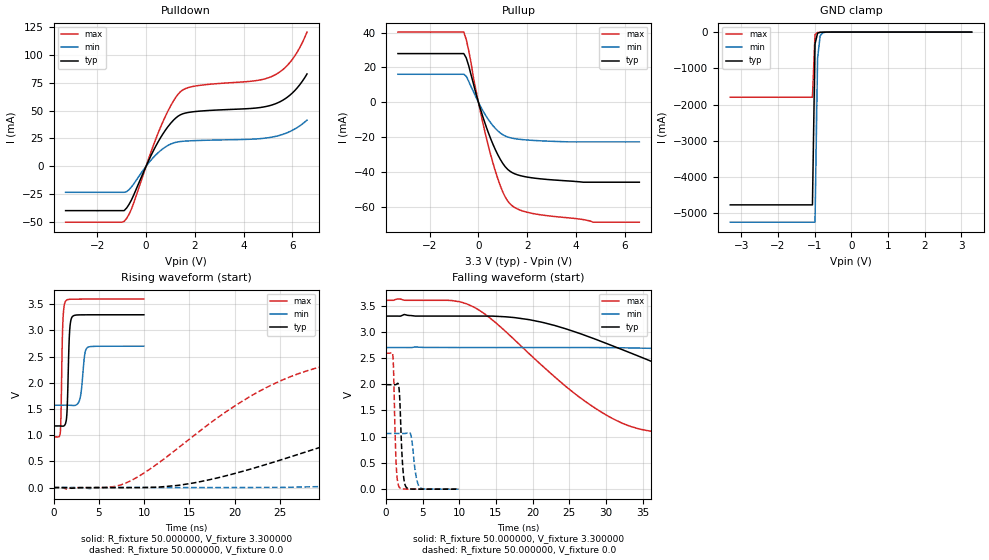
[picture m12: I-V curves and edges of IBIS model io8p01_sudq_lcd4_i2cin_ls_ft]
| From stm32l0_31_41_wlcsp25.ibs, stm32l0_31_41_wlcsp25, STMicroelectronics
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|   Model io8p01_sudq_lcd4_i2cin_ls_ft
[Model]  io8p01_sudq_lcd4_i2cin_ls_ft
Model_type I/O
Polarity   Non-Inverting
Enable   Active-Low
Vinl =   0.990000V
Vinh =   2.310000V
Vmeas =  1.650000V
Cref =   50.000000pF
Rref =   100.000000M
Vref =   0.0V
C_comp   2.499500pF   2.460800pF   2.557800pF
[Temperature Range]   25.000000   0.125000k   -40.000000
[Pullup Reference]   3.300000V   2.700000V   3.600000V
[Pulldown Reference]   0.0V   0.0V   0.0V
[POWER Clamp Reference]   3.300000V   2.700000V   3.600000V
[GND Clamp Reference]   0.0V   0.0V   0.0V
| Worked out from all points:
|   slope of the pulldown table from 0 to 0.495 V, typ, clamps not added: 22.6 ohm
|   slope of the pullup table from 0 to 0.495 V, typ, clamps not added: 23.9 ohm
|   GND clamp passes 1 mA (typ) near -0.64 V on its own axis
|   rising waveform, R_fixture 50.000000, V_fixture 3.300000: 20-80 % time 216ps typ, 364ps min, 176ps max; typ from 1.18 V to 3.3 V
|   rising waveform, R_fixture 50.000000, V_fixture 0.0: 20-80 % time 27.1ns typ, 59.7ns min, 13.6ns max; typ from 0 V to 1.99 V
|   falling waveform, R_fixture 50.000000, V_fixture 3.300000: 20-80 % time 24.2ns typ, 53.5ns min, 13.3ns max; typ from 3.3 V to 1.18 V
|   falling waveform, R_fixture 50.000000, V_fixture 0.0: 20-80 % time 383ps typ, 552ps min, 305ps max; typ from 1.99 V to 0 V
[Pulldown]
|Voltage   I(typ)   I(min)   I(max)
-3.3V     -39.83mA   -23.37mA   -50.2mA
-900mV    -39.83mA   -23.37mA   -49.53mA
-600mV    -30.28mA   -18.59mA   -38.45mA
500mV     22.11mA    12.28mA    30.1mA
1V        38.33mA    19.81mA    53.88mA
1.4V      46.1mA     22.18mA    66.72mA
2V        49.07mA    23.01mA    71.93mA
4.4V      52.05mA    24.38mA    76.53mA
5.2V      55.25mA    26.3mA     81.02mA
5.6V      59.18mA    28.57mA    86.57mA
6V        65.78mA    32.24mA    95.96mA
6.6V      82.83mA    41.41mA    120.4mA
[Pullup]
|Voltage   I(typ)   I(min)   I(max)
-3.3V     27.97mA    16.08mA    40.34mA
-600mV    27.97mA    16.08mA    40.34mA
-400mV    21.06mA    12.09mA    29.9mA
-200mV    10.4mA     5.946mA    13.84mA
200mV     -9.115mA   -5.294mA   -12.98mA
600mV     -24.29mA   -13.56mA   -35.12mA
1V        -35.2mA    -18.69mA   -51.63mA
1.2V      -38.62mA   -20mA      -56.79mA
1.4V      -40.6mA    -20.72mA   -59.71mA
2.2V      -43.48mA   -21.92mA   -63.91mA
4.7V      -46.01mA   -22.8mA    -69mA
6.6V      -46.01mA   -22.8mA    -69mA
[GND_clamp]
|Voltage   I(typ)   I(min)   I(max)
-3.3V     -4.766A    -5.244A    -1.797A
-1.06V    -4.766A    -5.244A    -1.797A
-990mV    -326.4mA   -5.244A    -67.85mA
-920mV    -28.83mA   -721.7mA   -11.08mA
-850mV    -6.686mA   -104.1mA   -6.707mA
-780mV    -3.552mA   -17.28mA   -4.326mA
-500mV    -59.41uA   -172uA     -34.91uA
3.28V     0A         0A         0A
[POWER_clamp]
|Voltage   I(typ)   I(min)   I(max)
-3.28V    0A         0A         0A
0V        0A         0A         0A
[Ramp]
| variable   typ   min   max
dV/dt_r  1.19496/27.05921n   0.63564/59.66275n   1.55568/13.54533n
dV/dt_f  1.27416/24.17291n   0.67062/53.43302n   1.57856/13.27860n
R_load = 50.000000
[Rising Waveform]
R_fixture= 50.000000
V_fixture= 3.300000
V_fixture_min= 2.700000
V_fixture_max= 3.600000
|time   V(typ)   V(min)   V(max)
0s        1.176V     1.573V     969.1mV
740.7ps   1.176V     1.573V     1.04V
1.021ns   1.173V     1.573V     3.119V
1.341ns   1.233V     1.574V     3.562V
1.502ns   1.5V       1.574V     3.586V
1.782ns   2.998V     1.572V     3.596V
2.082ns   3.266V     1.569V     3.598V
2.903ns   3.298V     1.688V     3.599V
3.724ns   3.299V     2.672V     3.599V
9.97ns    3.3V       2.7V       3.6V
[Rising Waveform]
R_fixture= 50.000000
V_fixture= 0.0
V_fixture_min= 0.0
V_fixture_max= 0.0
|time   V(typ)   V(min)   V(max)
0s        -596.2nV   -2.465uV   -306.5nV
8.008ns   -451.4uV   -168.4uV   88.51mV
15.52ns   89.78mV    -154.7uV   994.8mV
25.03ns   524.6mV    2.952mV    2.036V
31.03ns   855.4mV    24.69mV    2.367V
38.54ns   1.216V     69.74mV    2.517V
57.06ns   1.748V     273.4mV    2.584V
81.58ns   1.946V     586.9mV    2.592V
146.6ns   1.991V     989.7mV    2.593V
249.2ns   1.992V     1.062V     2.593V
[Falling Waveform]
R_fixture= 50.000000
V_fixture= 3.300000
V_fixture_min= 2.700000
V_fixture_max= 3.600000
|time   V(typ)   V(min)   V(max)
0s        3.3V       2.7V       3.6V
12.01ns   3.3V       2.7V       3.471V
19.52ns   3.232V     2.7V       2.584V
28.53ns   2.861V     2.7V       1.544V
33.53ns   2.587V     2.692V     1.188V
39.04ns   2.274V     2.671V     1.06V
56.06ns   1.482V     2.524V     987.8mV
74.57ns   1.269V     2.272V     973.9mV
130.1ns   1.184V     1.712V     969.2mV
249.2ns   1.176V     1.573V     969.1mV
[Falling Waveform]
R_fixture= 50.000000
V_fixture= 0.0
V_fixture_min= 0.0
V_fixture_max= 0.0
|time   V(typ)   V(min)   V(max)
0s        1.992V     1.062V     2.593V
961ps     1.992V     1.062V     2.536V
1.401ns   1.996V     1.062V     490.4mV
1.802ns   1.912V     1.062V     44.08mV
2.282ns   465.2mV    1.061V     4.108mV
2.763ns   40.06mV    1.065V     1.489mV
3.423ns   2.595mV    1.022V     872uV
4.104ns   882.8uV    258.1mV    557.6uV
4.665ns   559.1uV    28.68mV    391.8uV
9.97ns    -596.2nV   -2.465uV   -306.5nV
